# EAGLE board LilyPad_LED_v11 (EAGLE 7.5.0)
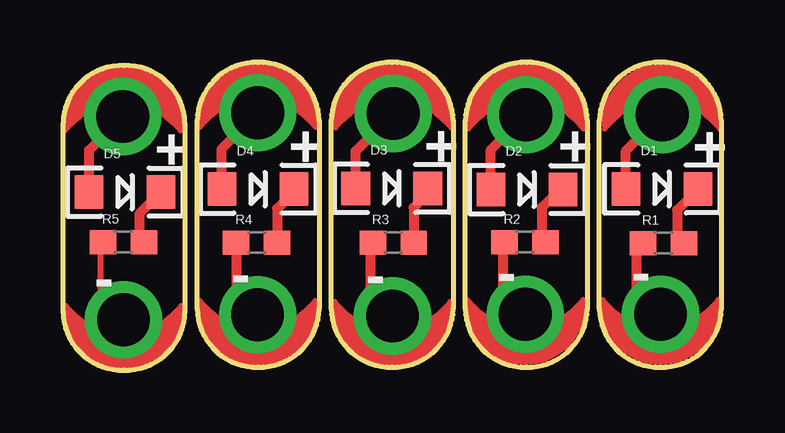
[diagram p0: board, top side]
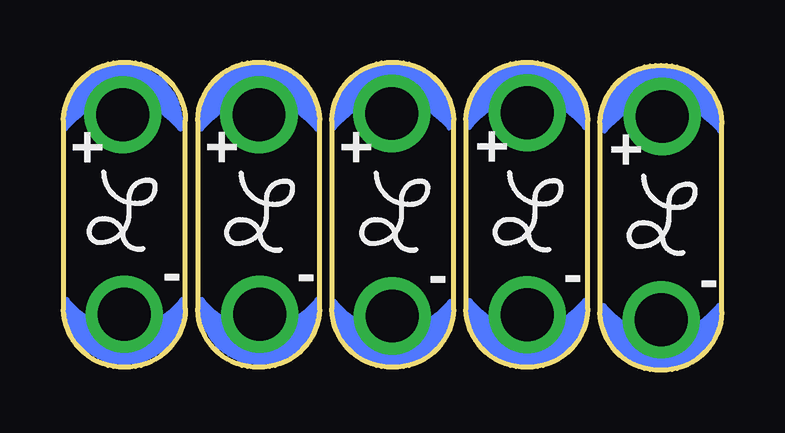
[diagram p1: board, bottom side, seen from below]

Size 27.43 x 12.83 mm. Coordinates in mm from the lower left corner, seen from the top.
Outline: 2.54,12.64 arc3 2.54,12.64
Outline: 2.54,0.06 arc3 2.54,0.06
Outline: 8.13,12.76 arc3 8.13,12.76
Outline: 13.71,12.76 arc3 13.72,12.76
Outline: 19.3,12.76 arc3 19.31,12.76
Outline: 5.08,10.29 arc90 2.54,12.7 arc90 0,10.29 0,2.41 arc90 2.54,0 arc90 5.08,2.41 5.08,10.29
Outline: 10.67,10.41 arc90 8.13,12.83 arc90 5.59,10.41 5.59,2.54 arc90 8.13,0.13 arc90 10.67,2.54 10.67,10.41
Outline: 16.26,10.41 arc90 13.72,12.83 arc90 11.18,10.41 11.18,2.54 arc90 13.72,0.13 arc90 16.26,2.54 16.26,10.41
Outline: 21.84,10.41 arc90 19.3,12.83 arc90 16.76,10.41 16.76,2.54 arc90 19.3,0.13 arc90 21.84,2.54 21.84,10.41
Outline: 27.43,10.41 arc90 24.89,12.83 arc90 22.35,10.41 22.35,2.54 arc90 24.89,0.13 arc90 27.43,2.54 27.43,10.41
Copper layers (1*16): Top 0.035mm / dielectric 1.5mm / Bottom 0.035mm
Design rules "SparkFun-2-layer-STANDARD": minimum track width 10mil, minimum drill 20mil, track to track 10mil, track to pad 8mil, pad to pad 8mil, via to via 10mil, smd to smd 8mil, copper to edge 8mil, drill to drill 8mil, minimum pad ring 10mil, minimum via ring 10mil, stop-mask expansion 4mil, vias tented up to drill 25mil, thermal gap 10mil

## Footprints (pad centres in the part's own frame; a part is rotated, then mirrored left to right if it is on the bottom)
LED-1206 = smd 1.2 x 1.4: A -1.5,0; C 1.5,0
PETAL-SMALL-2SIDE = drill 2.2: 1 0,0
0603-RES = smd 1.1 x 1: 1 -0.85,0; 2 0.85,0

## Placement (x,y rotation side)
D1  WHITE  [LED-1206]  24.96,7.55 0 top
D2  WHITE  [LED-1206]  19.33,7.53 0 top
D3  WHITE  [LED-1206]  13.7,7.57 0 top
D4  WHITE  [LED-1206]  8.12,7.54 0 top
D5  WHITE  [LED-1206]  2.58,7.42 0 top
FRAME1  FRAME-LETTER  [CREATIVE_COMMONS]  not placed on the board
LED+1  SEWTAP6  [PETAL-SMALL-2SIDE]  24.96,10.64 180 top
LED+2  SEWTAP6  [PETAL-SMALL-2SIDE]  19.29,10.64 180 top
LED+3  SEWTAP6  [PETAL-SMALL-2SIDE]  13.76,10.7 180 top
LED+4  SEWTAP6  [PETAL-SMALL-2SIDE]  8.12,10.72 180 top
LED+5  SEWTAP6  [PETAL-SMALL-2SIDE]  2.49,10.57 180 top
LED-1  SEWTAP6  [PETAL-SMALL-2SIDE]  24.89,2.34 0 top
LED-2  SEWTAP6  [PETAL-SMALL-2SIDE]  19.26,2.34 0 top
LED-3  SEWTAP6  [PETAL-SMALL-2SIDE]  13.73,2.26 0 top
LED-4  SEWTAP6  [PETAL-SMALL-2SIDE]  8.11,2.31 0 top
LED-5  SEWTAP6  [PETAL-SMALL-2SIDE]  2.52,2.11 0 top
R1  150  [0603-RES]  25.02,5.29 0 top
R2  150  [0603-RES]  19.25,5.33 0 top
R3  150  [0603-RES]  13.76,5.31 0 top
R4  150  [0603-RES]  8.06,5.31 0 top
R5  150  [0603-RES]  2.52,5.33 0 top
U$1  [LOGO-L]  24.99,6.64 0 bottom
U$2  [LOGO-L]  19.26,6.6 0 bottom
U$3  [LOGO-L]  13.63,6.6 0 bottom
U$4  [LOGO-L]  8.07,6.61 0 bottom
U$5  [LOGO-L]  2.49,6.47 0 bottom
U$6  REVISION  [REVISION]  not placed on the board

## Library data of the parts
D1-D5 = SparkFun-LED; PROD_ID: DIO-09955
FRAME1 U$6 = SparkFun-Aesthetics
LED+1-LED+5 LED-1-LED-5 U$1-U$5 = LilyPad-Wearables
R1-R5 = SparkFun-Resistors; PROD-ID: 13326

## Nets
1: D1.A LED+1.1
2: D1.C R1.2
3: LED-1.1 R1.1
4: D2.A LED+2.1
5: D2.C R2.2
6: LED-2.1 R2.1
7: D3.A LED+3.1
8: D3.C R3.2
9: LED-3.1 R3.1
10: D4.A LED+4.1
11: D4.C R4.2
12: LED-4.1 R4.1
13: D5.A LED+5.1
14: D5.C R5.2
15: LED-5.1 R5.1

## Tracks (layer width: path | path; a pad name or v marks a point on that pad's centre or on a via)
1
  Top 0.406: D1.A 23.46,9.13 LED+1.1
2
  Top 0.406: D1.C 26.46,7.54 25.58,6.67 25.58,5.57 R1.2
3
  Top 0.406: LED-1.1 23.91,3.32 23.91,5.03 R1.1
4
  Top 0.406: D2.A 17.83,9.19 LED+2.1
5
  Top 0.406: D2.C 20.7,7.53 19.95,6.77 19.95,5.48 R2.2
6
  Top 0.406: LED-2.1 18.34,3.25 18.34,5.28 R2.1
7
  Top 0.406: D3.A 12.2,9.13 LED+3.1
8
  Top 0.406: D3.C 15.2,7.35 14.61,6.77 R3.2
9
  Top 0.254: 12.81,5.21 R3.1
  Top 0.406: LED-3.1 12.81,3.17 12.81,5.21
10
  Top 0.406: D4.A 6.62,9.23 LED+4.1
11
  Top 0.406: D4.C 9.62,7.43 8.92,6.73 R4.2
12
  Top 0.406: R4.1 7.21,3.2 LED-4.1
13
  Top 0.406: D5.A 1.08,9.17 LED+5.1
14
  Top 0.406: D5.C 3.18,6.52 3.18,5.52 R5.2
15
  Top 0.254: 1.57,3.06 1.57,5.23 R5.1
  Top 0.406: 1.57,3.06 LED-5.1

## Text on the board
tPlace: + | + | + | + | + | - | - | - | - | -
bPlace: + | + | + | + | + | - | - | - | - | -
Measures: All Units Inches
tDocu: Board Thickness: 0.032" | Purple Solder Mask | L. Buechley | M. West | v11

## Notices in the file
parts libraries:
SparkFun-LED: Licensing: Creative Commons ShareAlike 4.0 International - https://creativecommons.org/licenses/by-sa/4.0
SparkFun-Aesthetics: Released under the Creative Commons Attribution Share-Alike 4.0 License
SparkFun-Aesthetics: https://creativecommons.org/licenses/by-sa/4.0
